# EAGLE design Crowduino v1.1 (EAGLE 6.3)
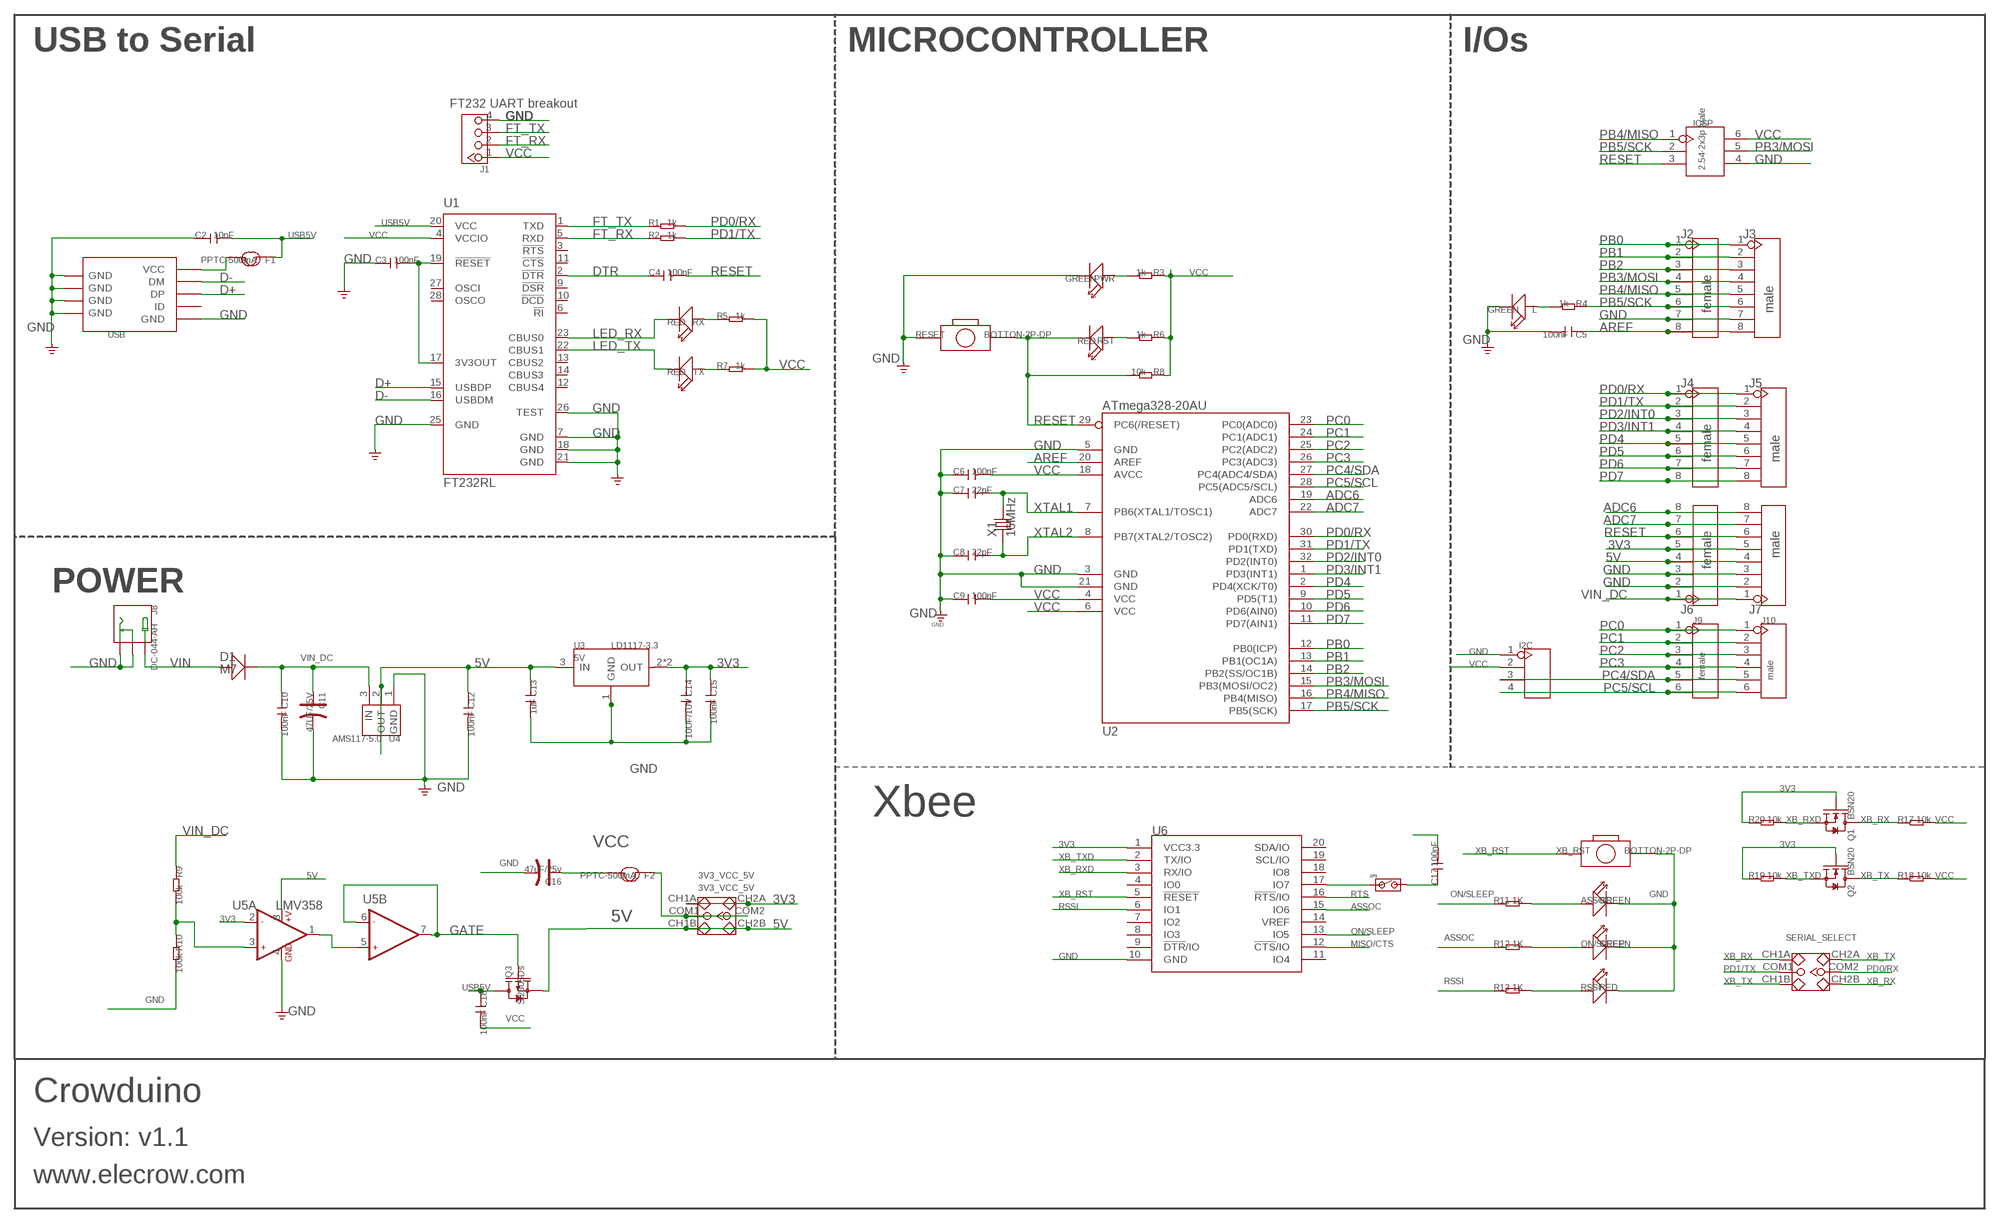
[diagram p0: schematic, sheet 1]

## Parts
3V3_VCC_5V  3V3_VCC_5V  SWITCH-2CH-6P  [6P-2CH-2.54-7.6X3.0]
ASSOC  GREEN  LED'0603'  [LED-0603]
C2  10nF  C-0603  [C0603]
C3  100nF  C-0603  [C0603]
C4  100nF  C-0603  [C0603]
C5  100nF  C-0603  [C0603]
C6  100nF  C-0603  [C0603]
C7  22pF  C-0603  [C0603]
C8  22pF  C-0603  [C0603]
C9  100nF  C-0603  [C0603]
C10  100nF  C-0603  [C0603]
C11  47UF/25V  CAP-ELECTRO-C  [ELECTRO-SMD-C-6MM]
C12  100nF  C-0603  [C0603]
C13  1uF  C-0603  [C0603]
C14  10UF/10V  C-0805  [C0805]
C15  100nF  C-0603  [C0603]
C16  47uF/25v  CAP-ELECTRO-C  [ELECTRO-SMD-C-6MM]
C17  100nF  C-0603  [C0603]
C18  100nF  C-0603  [C0603]
D1  M7  D-SMA  [D2010]
F1  PPTC-500mA  FUSE  [1206@1]
F2  PPTC-500mA  FUSE  [1206@1]
I2C  HEADER-4P-60/35MIL  [4P-65/35MIL]
ICSP  2.54-2x3p male  HEADER-2X3P-2.54  [2X3P-2.54]
J1  CK_1X4_DD  [CK_1X4]
J2  female  HEADER-8P-65/35MIL  [8P-2.54-65/35MIL]
J3  male  HEADER-8P-65/35MIL  [8P-2.54-65/35MIL]
J4  female  HEADER-8P-65/35MIL  [8P-2.54-65/35MIL]
J5  male  HEADER-8P-65/35MIL  [8P-2.54-65/35MIL]
J6  female  HEADER-8P-65/35MIL  [8P-2.54-65/35MIL]
J7  male  HEADER-8P-65/35MIL  [8P-2.54-65/35MIL]
J8  DC-044-AH  DC-044  [DC-404]
J9  female  HEADER-6P-65/35MIL  [6P-2.54-65/35MIL]
J10  male  HEADER-6P-65/35MIL  [6P-2.54-65/35MIL]
JP1  CPT_SMD_JP_SW  [CPT_SMD_JP_SW]
L  GREEN  LED'0603'  [LED-0603]
ON/SLEEP  GREEN  LED'0603'  [LED-0603]
PWR  GREEN  LED'0603'  [LED-0603]
Q1  BSN20  MOSFET-N'SOT23'  [SOT23]
Q2  BSN20  MOSFET-N'SOT23'  [SOT23]
Q3  Si2305Ds  MOSFET-P'SI2323CDS/SI2305DS<BR>'  [SOT23@1]
R1  1k  R-0603  [R0603]
R2  1k  R-0603  [R0603]
R3  1k  R-0603  [R0603]
R4  1k  R-0603  [R0603]
R5  1k  R-0603  [R0603]
R6  1k  R-0603  [R0603]
R7  1k  R-0603  [R0603]
R8  10k  R-0603  [R0603]
R9  100k  R-0603  [R0603]
R10  100k  R-0603  [R0603]
R11  1K  R-0603  [R0603]
R12  1K  R-0603  [R0603]
R13  1K  R-0603  [R0603]
R17  10k  R-0603  [R0603]
R18  10k  R-0603  [R0603]
R19  10k  R-0603  [R0603]
R20  10k  R-0603  [R0603]
RESET  BOTTON-2P-DP  BOTTON-2P-90D  [2P-7.62X3.56-90D]
RSSI  RED  LED'0603'  [LED-0603]
RST  RED  LED'0603'  [LED-0603]
RX  RED  LED'0603'  [LED-0603]
SERIAL_SELECT  3V3_VCC_5V  SWITCH-2CH-6P  [6P-2CH-2.54-7.6X3.0]
TX  RED  LED'0603'  [LED-0603]
U1  FT232RL  [SSOP28]
U2  ATmega328-20AU  ATMEGA168  [TQFP32]
U3  LD1117-3.3  LD1117'SOT89'  [SOT89]
U4  AMS117-5.0  AMS1117SOT223  [SOT-223@1]
U5  LMV358  [SO08]
U6  BEE-OPENBEE  [20-DIP-2.0-W/-SILK]
USB  USB-MINIUSB-5P-STRONG  [MINI-SMD-5P]
X1  16MHz  CRYSTAL-HC49S  [HC49/S]
XB_RST  BOTTON-2P-DP  BOTTON-2P-90D  [2P-7.62X3.56-90D]

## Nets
3V3: 3V3_VCC_5V.CH1A 3V3_VCC_5V.CH2A C14.1 C15.1 J6.5 J7.5 Q1.1(G) Q2.1(G) R19.1 R20.1 U3.2(OUT) U3.4(OUT) U5.2(A:-IN1) U6.1(VCC3.3)
5V [usbvcc]: 3V3_VCC_5V.CH1B 3V3_VCC_5V.CH2B C12.1 C13.1 J6.4 J7.4 Q3.2(S) U3.3(IN) U4.2(OUT) U4.TER(TAB) U5.8(A:+V)
ADC6: J6.8 J7.8 U2.19(ADC6)
ADC7: J6.7 J7.7 U2.22(ADC7)
AREF: C5.1 J2.8 J3.8 U2.20(AREF)
ASSOC: R12.1 U6.15(IO6)
D+: U1.15(USBDP) USB.3(DP)
D-: U1.16(USBDM) USB.2(DM)
DTR: C4.1 U1.2(!DTR)
FT_RX: J1.2 R2.1 U1.5(RXD)
FT_TX: J1.3 R1.1 U1.1(TXD)
GATE: Q3.1(G) U5.6(B:-IN2) U5.7(B:OUT2)
GND: ASSOC.- C2.1 C3.1 C5.2 C6.1 C7.1 C8.1 C9.1 C10.2 C11.- C12.2 C13.2 C14.2 C15.2 C16.- I2C.1 ICSP.4 J1.4 J2.7 J3.7 J6.2 J6.3 J7.2 J7.3 J8.- J8.CDN L.- ON/SLEEP.- PWR.- R10.2 RESET.P$1 RSSI.- U1.7(GND) U1.18(GND) U1.21(GND) U1.25(GND) U1.26(TEST) U2.3(GND) U2.5(GND) U2.21(GND) U3.1(GND) U4.1(GND) U5.4(A:GND) U6.10(GND) USB.5(GND) USB.GND@1(GND) USB.GND@2(GND) USB.GND@3(GND) USB.GND@4(GND) XB_RST.P$2
LED_RX: RX.- U1.23(CBUS0)
LED_TX: TX.- U1.22(CBUS1)
MISO/CTS: U6.12(!CTS!/IO)
N$1: U5.1(A:OUT1) U5.5(B:+IN2)
N$2: F1.2 USB.1(VCC)
N$3: L.+ R4.2
N$4: 3V3_VCC_5V.COM1 3V3_VCC_5V.COM2 F2.1
N$5: JP1.1 U6.17(IO7)
N$6: C3.2 U1.17(3V3OUT) U1.19(!RESET)
N$7: PWR.+ R3.2
N$8: C17.1 JP1.2
N$9: R13.2 RSSI.+
N$11: ON/SLEEP.+ R12.2
N$12: ASSOC.+ R11.2
N$14: R9.2 R10.1 U5.3(A:+IN1)
N$17: R6.2 RST.+
N$31: R5.1 RX.+
N$32: R7.1 TX.+
ON/SLEEP: R11.1 U6.13(IO5)
PB0: J2.1 J3.1 U2.12(PB0(ICP))
PB1: J2.2 J3.2 U2.13(PB1(OC1A))
PB2: J2.3 J3.3 U2.14(PB2(SS/OC1B))
PB3/MOSI: ICSP.5 J2.4 J3.4 U2.15(PB3(MOSI/OC2))
PB4/MISO: ICSP.1 J2.5 J3.5 U2.16(PB4(MISO))
PB5/SCK: ICSP.2 J2.6 J3.6 R4.1 U2.17(PB5(SCK))
PC0: J9.1 J10.1 U2.23(PC0(ADC0))
PC1: J9.2 J10.2 U2.24(PC1(ADC1))
PC2: J9.3 J10.3 U2.25(PC2(ADC2))
PC3: J9.4 J10.4 U2.26(PC3(ADC3))
PC4/SDA: I2C.3 J9.5 J10.5 U2.27(PC4(ADC4/SDA))
PC5/SCL: I2C.4 J9.6 J10.6 U2.28(PC5(ADC5/SCL))
PD0/RX: J4.1 J5.1 R1.2 SERIAL_SELECT.COM2 U2.30(PD0(RXD))
PD1/TX: J4.2 J5.2 R2.2 SERIAL_SELECT.COM1 U2.31(PD1(TXD))
PD2/INT0: J4.3 J5.3 U2.32(PD2(INT0))
PD3/INT1: J4.4 J5.4 U2.1(PD3(INT1))
PD4: J4.5 J5.5 U2.2(PD4(XCK/T0))
PD5: J4.6 J5.6 U2.9(PD5(T1))
PD6: J4.7 J5.7 U2.10(PD6(AIN0))
PD7: J4.8 J5.8 U2.11(PD7(AIN1))
RESET: C4.2 C17.2 ICSP.3 J6.6 J7.6 R8.2 RESET.P$2 RST.- U2.29(PC6(/RESET))
RSSI: R13.1 U6.6(IO1)
RTS: U6.16(!RTS!/IO)
USB5V: C2.2 C18.1 F1.1 Q3.3(D) U1.20(VCC)
VCC: C6.2 C9.2 C16.+ C18.2 F2.2 I2C.2 ICSP.6 J1.1 R3.1 R5.2 R6.1 R7.2 R8.1 R17.2 R18.2 U1.4(VCCIO) U2.4(VCC) U2.6(VCC) U2.18(AVCC)
VIN: D1.+ J8.+
VIN_DC: C10.1 C11.+ D1.- J6.1 J7.1 R9.1 U4.3(IN)
XB_RST: U6.5(!RESET) XB_RST.P$1
XB_RX: Q1.3(D) R17.1 SERIAL_SELECT.CH1A SERIAL_SELECT.CH2B
XB_RXD: Q1.2(S) R20.2 U6.3(RX/IO)
XB_TX: Q2.3(D) R18.1 SERIAL_SELECT.CH1B SERIAL_SELECT.CH2A
XB_TXD: Q2.2(S) R19.2 U6.2(TX/IO)
XTAL1: C7.2 U2.7(PB6(XTAL1/TOSC1)) X1.2
XTAL2: C8.2 U2.8(PB7(XTAL2/TOSC2)) X1.1
Unconnected: U1.3(!RTS) U1.6(!RI) U1.9(!DSR) U1.10(!DCD) U1.11(!CTS) U1.12(CBUS4) U1.13(CBUS2) U1.14(CBUS3) U1.27(OSCI) U1.28(OSCO) U6.4(IO0) U6.7(IO2) U6.8(IO3) U6.9(!DTR!/IO) U6.11(IO4) U6.14(VREF) U6.18(IO8) U6.19(SCL/IO) U6.20(SDA/IO) USB.4(ID)

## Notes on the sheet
- USB to Serial | MICROCONTROLLER | I/Os
- FT232 UART breakout
- POWER
- Xbee
- Crowduino
- Version: v1.1
- www.elecrow.com

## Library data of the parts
3V3_VCC_5V SERIAL_SELECT = Discrete:SWITCH-2CH-6P
ASSOC L ON/SLEEP PWR RSSI RST RX TX = Discrete:LED*
C2-C10 C12-C15 C17 C18 = Discrete:C*: Ceramic Capacitors
C11 C16 = Discrete:CAP*: Electrolytic Capacitors,Tantalum Capacitors and Super Capacitors
D1 = Discrete:D*
F1 F2 = Discrete:FUSE
I2C = Connector:HEADER-4P
ICSP = Connector:HEADER-2X3P
J1 = CONNECTER:CK_1X4
J2-J7 = Connector:HEADER-8P
J8 = For_Test_Albert:DC-044
J9 J10 = Connector:HEADER-6P
JP1 = Elecrow_test:CPT_SMD_JP_SW
Q1 Q2 = Discrete:MOSFET-N: IRLL014: http://www.vishay.com/docs/91319/sihll014.pdf
Q3 = Discrete:MOSFET-P
R1-R13 R17-R20 = Discrete:R*
RESET XB_RST = Discrete:BOTTON-2P
U1 = IC_SMD:FT232R: Source: http://www.ftdichip.com/Documents/DataSheets/DS_FT232R_v104.pdf
U2 = IC:ATMEGA168
U3 = IC:LD1117: Low Drop Fixed And Adjustable Positive Voltage Regulators http://www.datasheetcatalog.org/datasheet/SGSThomsonMicroelectronics/mXuqtqv.pdf
U4 = IC:AMS1117
U5 = IC:LMV358
U6 = moudle:BEE-OPENBEE
USB = Connector:USB-MINIUSB-5P
X1 = Discrete:CRYSTAL*: CRYSTAL

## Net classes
0 default: clearance 0.152 mm
1 power: width 0.203 mm, drill 0.305 mm, clearance 0.203 mm
2 gnd: width 0.203 mm, drill 0.305 mm, clearance 0.203 mm
3 usbvcc: width 0.203 mm, drill 0.305 mm, clearance 0.203 mm

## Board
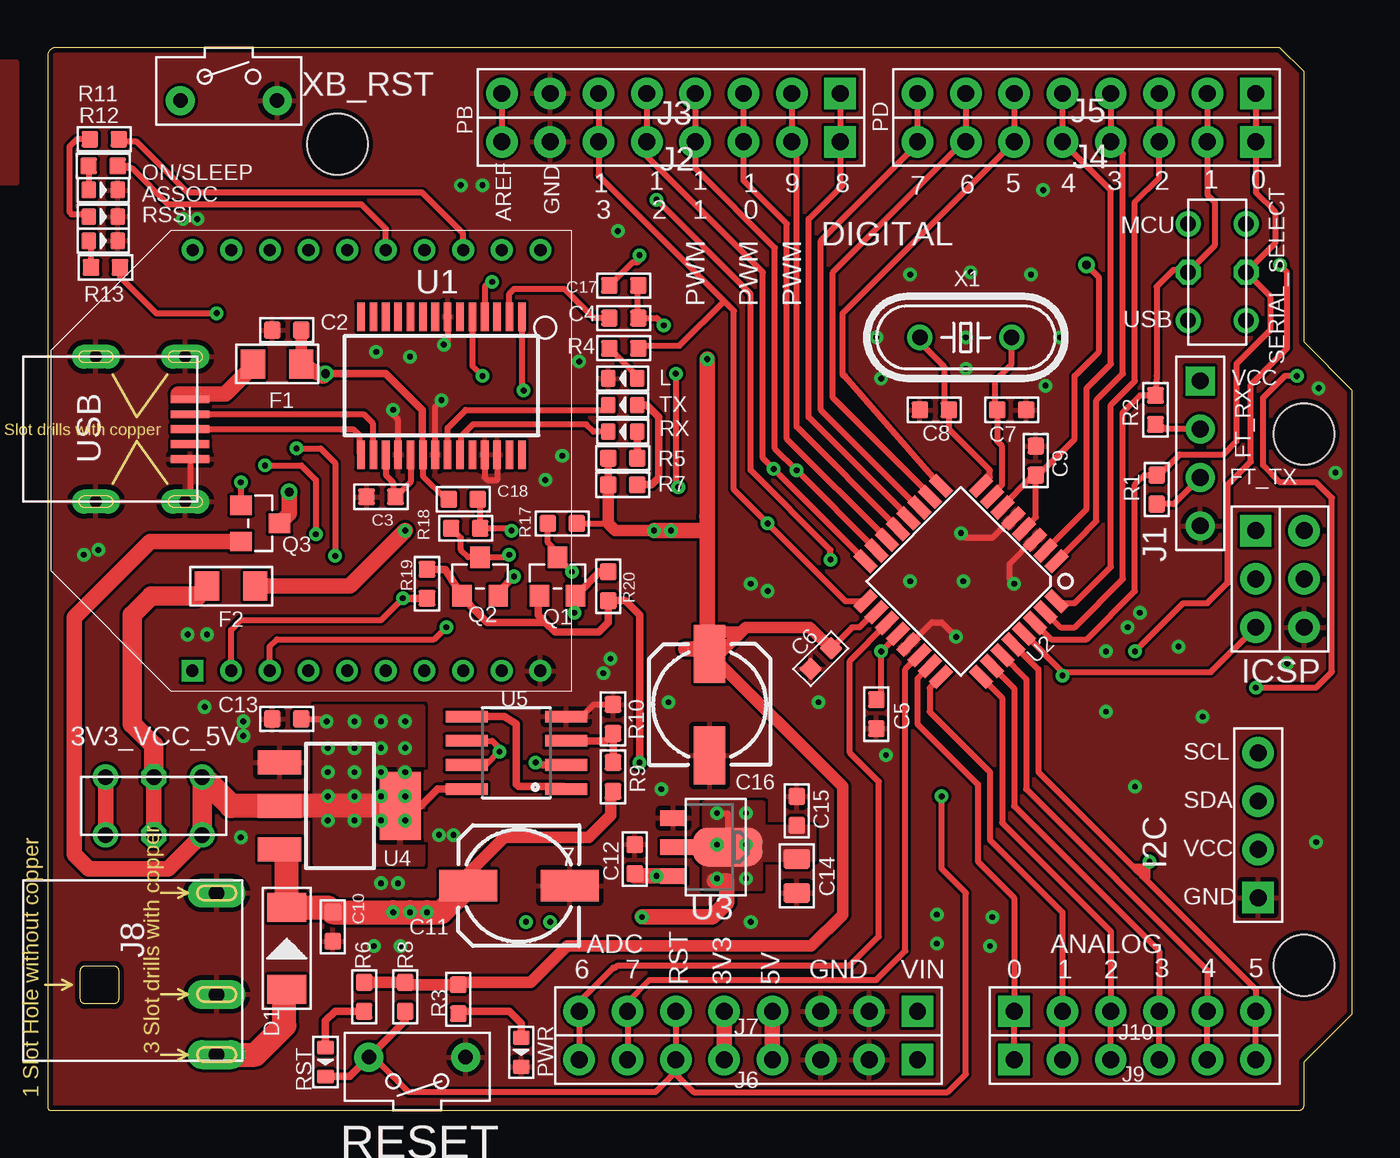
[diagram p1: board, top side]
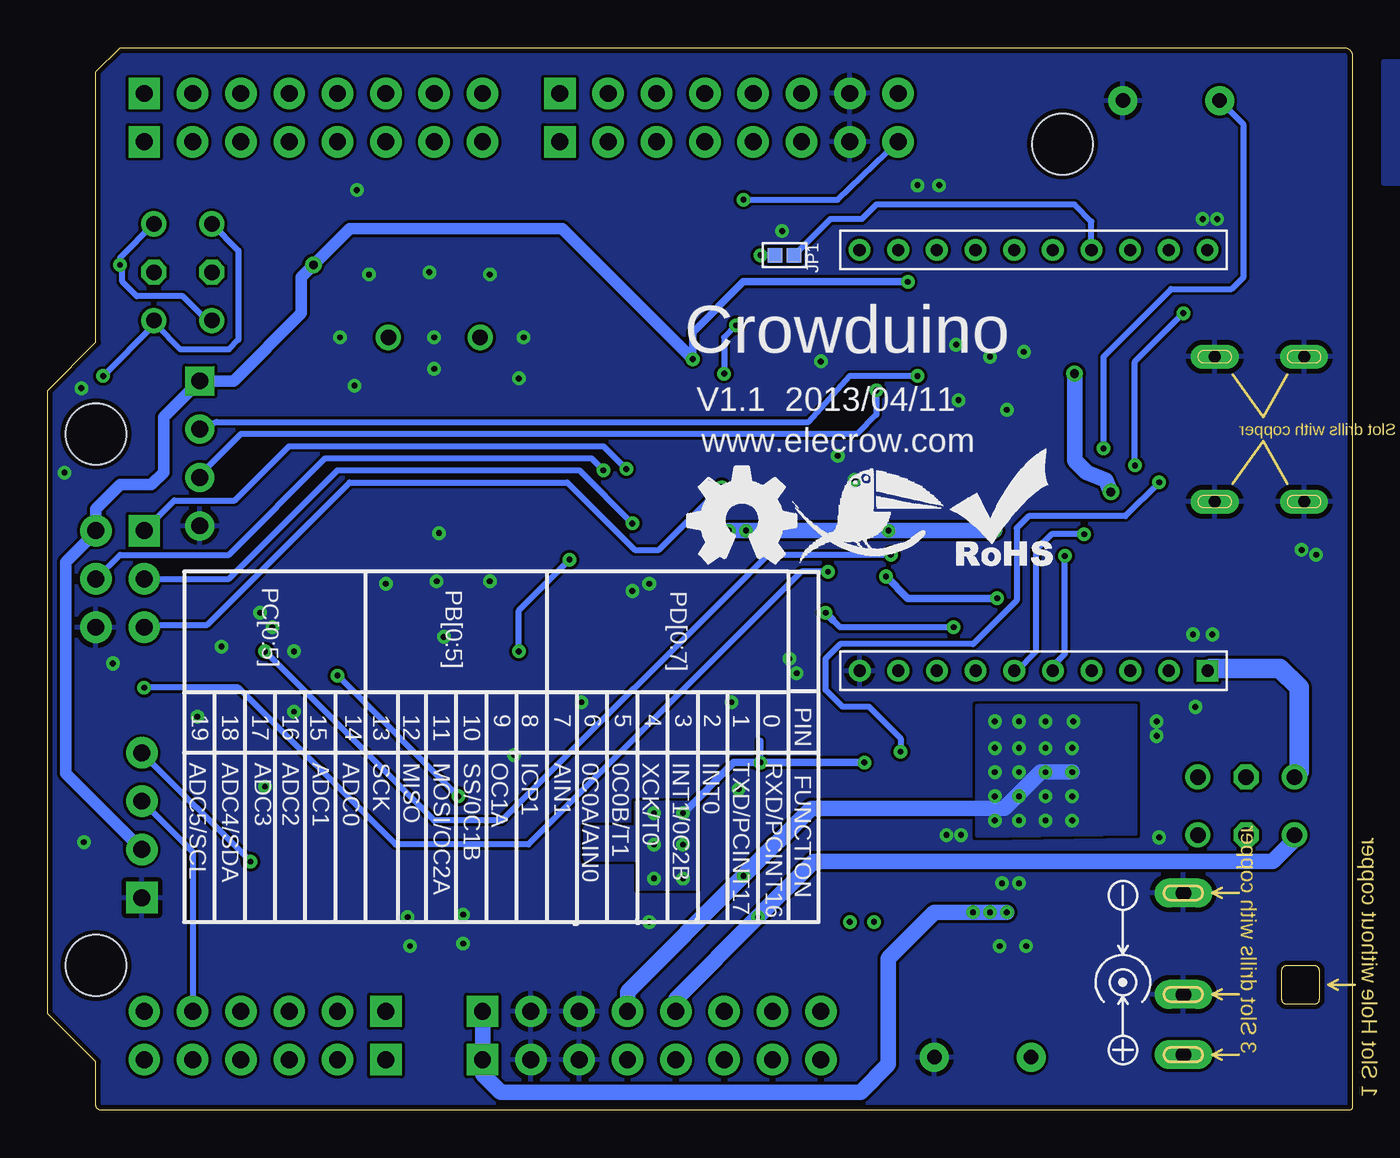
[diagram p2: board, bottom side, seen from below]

Size 68.58 x 55.88 mm. Coordinates in mm from the lower left corner, seen from the top.
Outline: 64.77,55.88 0.46,55.88 arc90 0,55.42 0,0.18 arc90 0.18,0 65.76,0 arc90 66.04,0.28 66.04,2.54 68.58,5.08 68.58,37.85 66.04,40.39 66.04,54.61 64.77,55.88
Copper layers (1*16): Top 0.035mm / dielectric 1.5mm / Bottom 0.035mm
Design rules "default *": minimum track width 10mil, minimum drill 12mil, track to track 6mil, track to pad 6mil, pad to pad 6mil, via to via 10mil, smd to smd 0mil, copper to edge 10mil, drill to drill 10mil, minimum pad ring 10mil, minimum via ring 8mil, stop-mask expansion 2mil, vias tented up to drill 25mil, thermal gap 10mil
Holes 3.2 mm at 66.04,7.62 66.04,35.56 15.24,50.8

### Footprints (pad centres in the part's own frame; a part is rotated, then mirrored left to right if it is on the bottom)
6P-2CH-2.54-7.6X3.0 = drill 0.813 pad 1.27: CH1A -1.524,2.54; CH1B -1.524,-2.54; CH2A 1.524,2.54; CH2B 1.524,-2.54 | drill 0.813 pad 1.27 octagon: COM1 -1.524,0; COM2 1.524,0
LED-0603 = smd 0.762 x 0.889: + -0.762,0; - 0.762,0
C0603 = smd 0.889 x 0.889: 1 -0.762,0; 2 0.762,0
ELECTRO-SMD-C-6MM = smd 3.048 x 1.651: + 2.667,0; - -2.667,0
C0805 = smd 1.016 x 1.397: 1 -0.889,0; 2 0.889,0
D2010 = smd 1.524 x 2.032: + -2.159,0; - 2.159,0
1206@1 = smd 1.27 x 1.524: 1 -1.27,0; 2 1.27,0
4P-65/35MIL = drill 0.889 pad 1.651 square: 1 0,3.81 | drill 0.889 pad 1.651: 2 0,1.27; 3 0,-1.27; 4 0,-3.81
2X3P-2.54 = drill 0.889 pad 1.651 square: 1 -1.27,2.54 | drill 0.889 pad 1.651: 2 -1.27,0; 3 -1.27,-2.54; 4 1.27,-2.54; 5 1.27,0; 6 1.27,2.54
CK_1X4 = drill 0.889 pad 1.524 square: 1 0,3.81 | drill 0.889 pad 1.524: 2 0,1.27; 3 0,-1.27; 4 0,-3.81
8P-2.54-65/35MIL = drill 0.889 pad 1.651 square: 1 0,8.89 | drill 0.889 pad 1.651: 2 0,6.35; 3 0,3.81; 4 0,1.27; 5 0,-1.27; 6 0,-3.81; 7 0,-6.35; 8 0,-8.89
DC-404 = drill 0.813 pad 1.524 long: + 3.175,10.16; - -5.334,10.16; CDN 0,10.16
6P-2.54-65/35MIL = drill 0.889 pad 1.651 square: 1 0,6.35 | drill 0.889 pad 1.651: 2 0,3.81; 3 0,1.27; 4 0,-1.27; 5 0,-3.81; 6 0,-6.35
CPT_SMD_JP_SW = smd 0.762 x 0.762: 1 0,0.508; 2 0,-0.508
SOT23 = smd 1.016 x 1.143: 1 -0.95,-1.016; 2 0.95,-1.016; 3 0,1.016
SOT23@1 = smd 1.016 x 1.143: 1 -0.95,-1.016; 2 0.95,-1.016; 3 0,1.016
R0603 = smd 0.889 x 0.889: 1 -0.762,0; 2 0.762,0
2P-7.62X3.56-90D = drill 0.762 pad 1.524: P$1 0,2.54; P$2 0,-2.54
SSOP28 = smd 0.4 x 1.5: 1 -4.225,-3.625; 2 -3.575,-3.625; 3 -2.925,-3.625; 4 -2.275,-3.625; 5 -1.625,-3.625; 6 -0.975,-3.625; 7 -0.325,-3.625; 8 0.325,-3.625; 9 0.975,-3.625; 10 1.625,-3.625; 11 2.275,-3.625; 12 2.925,-3.625; 13 3.575,-3.625; 14 4.225,-3.625; 15 4.225,3.625; 16 3.575,3.625; 17 2.925,3.625; 18 2.275,3.625; 19 1.625,3.625; 20 0.975,3.625; 21 0.325,3.625; 22 -0.325,3.625; 23 -0.975,3.625; 24 -1.625,3.625; 25 -2.275,3.625; 26 -2.925,3.625; 27 -3.575,3.625; 28 -4.225,3.625
TQFP32 = smd 1.27 x 0.559: 1 -4.293,2.8; 2 -4.293,2; 3 -4.293,1.2; 4 -4.293,0.4; 5 -4.293,-0.4; 6 -4.293,-1.2; 7 -4.293,-2; 8 -4.293,-2.8; 17 4.293,-2.8; 18 4.293,-2; 19 4.293,-1.2; 20 4.293,-0.4; 21 4.293,0.4; 22 4.293,1.2; 23 4.293,2; 24 4.293,2.8 | smd 0.559 x 1.27: 9 -2.8,-4.293; 10 -2,-4.293; 11 -1.2,-4.293; 12 -0.4,-4.293; 13 0.4,-4.293; 14 1.2,-4.293; 15 2,-4.293; 16 2.8,-4.293; 25 2.8,4.293; 26 2,4.293; 27 1.2,4.293; 28 0.4,4.293; 29 -0.4,4.293; 30 -1.2,4.293; 31 -2,4.293; 32 -2.8,4.293
SOT89 = smd 0.8 x 1.4: 1 -1.524,-1.905; 3 1.524,-1.905 | smd 0.8 x 1.9: 2 0,-1.651 | smd 2.032 x 3.65: 4 0,0.94
SOT-223@1 = smd 1.27 x 2.286: 1 -2.286,-3.175; 2 0,-3.175; 3 2.286,-3.175 | smd 3.556 x 2.159: TER 0,3.175
SO08 = smd 0.61 x 2.21: 1 -1.905,-2.616; 2 -0.635,-2.616; 3 0.635,-2.616; 4 1.905,-2.616; 5 1.905,2.616; 6 0.635,2.616; 7 -0.635,2.616; 8 -1.905,2.616
20-DIP-2.0-W/-SILK = drill 0.635 pad 1.016 square: 1 0,0.008 | drill 0.635 pad 1.016: 2 0,-2.024; 3 0,-4.056; 4 0,-6.088; 5 0,-8.12; 6 0,-10.152; 7 0,-12.184; 8 0,-14.216; 9 0,-16.248; 10 0,-18.28; 11 22.123,-18.288; 12 22.123,-16.256; 13 22.123,-14.224; 14 22.123,-12.192; 15 22.123,-10.16; 16 22.123,-8.128; 17 22.123,-6.096; 18 22.123,-4.064; 19 22.123,-2.032; 20 22.123,0
MINI-SMD-5P = smd 2.032 x 0.406: 1 0.381,-1.575; 2 0.381,-0.787; 3 0.381,0; 4 0.381,0.787; 5 0.381,1.575 | drill 0.635 pad 1.27 long: GND@1 0.635,3.81; GND@2 5.334,3.81; GND@3 5.334,-3.81; GND@4 0.635,-3.81
HC49/S = drill 0.813: 1 -2.413,0; 2 2.413,0

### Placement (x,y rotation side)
3V3_VCC_5V  5.59,16 90 top
ASSOC  2.92,46.99 0 top
C2  12.57,41.02 0 top
C3  17.53,32.26 0 top
C4  30.29,41.66 0 top
C5  43.56,20.83 270 top
C6  40.64,23.75 45 top
C7  50.67,36.83 180 top
C8  46.61,36.83 0 top
C9  51.94,34.16 270 top
C10  14.99,9.65 270 top
C11  24.77,11.81 180 top
C12  30.86,13.21 90 top
C13  12.57,20.57 180 top
C14  39.37,12.32 270 top
C15  39.37,15.75 90 top
C16  34.8,21.34 90 top
C17  30.29,43.37 0 top
C18  21.84,32.13 0 top
D1  12.57,8.51 90 top
F1  12.06,39.24 180 top
F2  9.65,27.56 0 top
I2C  63.63,14.99 180 top
ICSP  64.77,27.94 0 top
J1  60.58,34.54 0 top
J2  32.77,50.93 270 top
J3  32.77,53.47 270 top
J4  54.61,50.93 270 top
J5  54.61,53.47 270 top
J6  36.83,2.67 270 top
J7  36.83,5.21 270 top
J8  -1.27,6.1 270 top
J9  57.15,2.67 90 top
J10  57.15,5.21 90 top
JP1  29.84,44.96 270 bottom
L  30.23,38.48 180 top
ON/SLEEP  2.92,48.39 0 top
PWR  24.89,3.05 270 top
Q1  26.8,28.07 0 top
Q2  22.73,28.07 0 top
Q3  11.18,30.86 270 top
R1  58.29,32.64 90 top
R2  58.23,36.83 90 top
R3  21.59,5.84 270 top
R4  30.29,40.07 180 top
R5  30.23,34.29 180 top
R6  16.64,5.97 270 top
R7  30.23,32.89 180 top
R8  18.8,5.97 270 top
R9  29.72,17.53 90 top
R10  29.72,20.57 90 top
R11  2.98,51.05 180 top
R12  2.92,49.66 180 top
R13  3.05,44.32 180 top
R17  27.05,30.86 0 top
R18  21.97,30.61 0 top
R19  19.94,27.69 270 top
R20  29.46,27.56 90 top
RESET  19.43,2.79 270 top
RSSI  2.92,45.72 0 top
RST  14.61,2.54 270 top
RX  30.23,35.69 180 top
SERIAL_SELECT  61.47,44.07 0 top
TX  30.23,37.08 180 top
U1  20.7,38.1 180 top
U2  48.01,27.81 225 top
U3  34.8,13.84 270 top
U4  15.37,16 270 top
U5  24.64,18.8 90 top
U6  7.62,23.11 90 top
U$1  [OSHW_FILLX200_NOTEXT]  34.92,28.77 0 bottom
U$2  [ELECROW4]  30.23,27.37 0 bottom
U$3  [ROHS_SILK]  19.05,31.05 0 bottom
USB  7.87,35.81 180 top
X1  48.26,40.64 0 top
XB_RST  9.53,53.09 90 top

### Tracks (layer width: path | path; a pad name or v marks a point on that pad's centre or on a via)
3V3  (via drill 0.3)
  Top 0.305: C14.1 39.37,13.27 39.43,13.21 | 39.37,15.24 C15.1 | v35.18,15.62 35.74,15.62 U3.4
  Top 0.406: v31.11,18.29 31.11,26.04 30.35,26.8 R20.1 | 26.16,25.65 25.78,26.04 25.78,26.98 Q1.1 | R19.1 20.89,28.45 Q2.1 22.29,26.48 23.11,25.65 26.16,25.65 | 26.16,25.65 26.67,25.15 28.96,25.15 29.46,25.65 R20.1 | 29.72,26.54 R20.1 | U5.2 26.04,18.16 v25.65,18.29
  Top 0.813: 3V3_VCC_5V.CH2A 3V3_VCC_5V.CH1A | U3.2 35.18,13.84 | v31.24,10.16 34.92,10.16 35.69,10.92 35.69,12.06 35.05,12.06 | J6.5 J7.5
  Bottom 0.305: 31.11,19.43 v31.11,18.29
  Bottom 0.406: v25.65,18.29 v31.11,18.29 32.51,18.29 v35.18,15.62
  Bottom 0.813: 3V3_VCC_5V.CH1A 3.05,14.22 4.19,13.08 28.32,13.08 v31.24,10.16 35.56,5.84 J7.5
  Bottom 1.016: 3V3_VCC_5V.CH2A 2.79,17.78 2.79,22.23 3.81,23.24 7.49,23.24 U6.1
  other vias: 35.18,13.97 35.18,12.19 36.7,12.19 36.7,15.62 36.7,13.97
  pour Bottom (isolate 0.254, no thermals): 34.54,16.13 34.54,11.68 37.47,11.68 37.47,13.21 40.26,13.21 40.26,14.86 37.59,14.86 37.59,16.13
  pour Top (isolate 0.254, no thermals): 34.54,16.13 34.54,11.68 37.47,11.68 37.47,13.21 40.26,13.21 40.26,14.86 37.59,14.86 37.59,16.13
5V  (via drill 0.3)
  Top 0.305: C13.1 14.54,20.57 v14.67,20.45
  Top 0.406: U5.8 21.89,16.76 21.77,16.89 20.51,16.89 19.62,16 U4.TER
  Top 0.813: U3.3 v32,12.32 30.99,12.32 | 30.86,12.32 30.99,12.32 | C12.1 30.99,12.32 | 3V3_VCC_5V.CH1B 6.35,12.7 2.16,12.7 1.4,13.46 1.4,25.91 5.4,29.91 Q3.2 | J6.4 J7.4
  Top 1.016: 3V3_VCC_5V.CH2B 3V3_VCC_5V.CH1B
  Top 1.27: U4.TER U4.2 9.65,16 3V3_VCC_5V.CH2B
  Bottom 0.813: v14.73,17.78 v16.13,17.78 16.38,17.78 18.29,15.88 28.45,15.88 v32,12.32 38.1,6.22 J7.4
  other vias: 14.73,19.05 16.13,19.05 17.53,19.05 18.8,19.05 18.8,20.45 17.53,20.45 16.13,20.45 14.73,15.24 16.13,15.24 14.73,16.51 16.13,16.51 17.53,17.78 18.8,17.78 17.53,16.51 18.8,16.51 17.53,15.24 18.8,15.24
  pour Bottom: 11.43,14.61 11.43,21.21 19.68,21.21 19.68,14.48
  pour Top: 14.1,21.21 19.68,21.21 19.68,12.95 14.1,12.95
ADC6
  Top 0.305: U2.19 42.16,23.62 42.16,18.8 43.69,17.27 43.69,9.14 42.16,7.62 29.97,7.62 29.84,7.49 29.72,7.49 27.94,5.71 J7.8 J6.8
ADC7
  Top 0.305: U2.22 45.09,23.2 45.09,8.38 43.56,6.86 31.62,6.86 30.48,5.71 J7.7 J6.7
AREF  (via drill 0.3)
  Top 0.305: C5.1 43.81,21.84 v43.81,24.13 44.69,25 U2.20 | v41.15,28.96 41.15,29.46 36.96,33.66 36.96,42.93 v32,47.88 | J3.8 J2.8
  Bottom 0.305: v43.81,24.13 43.81,26.29 v41.15,28.96 | v32,47.88 27.05,47.88 J2.8
ASSOC
  Top 0.305: 4.19,49.66 R12.1 3.94,49.53 4.45,49.53 6.35,47.62 16.51,47.62 17.78,46.35 U6.15
D+
  Top 0.305: USB.3 16.07,35.81 16.38,35.5 16.38,34.57 U1.15
D-
  Top 0.305: USB.2 16.61,36.6 17.08,36.13 17.08,34.52 U1.16
DTR
  Top 0.305: U1.2 24.28,42.95 24.51,43.18 27.18,43.18 28.7,41.66 C4.1
FT_RX  (via drill 0.3)
  Top 0.305: J1.2 58.8,35.81 R2.1 | U1.5 22.33,39.14 v22.86,38.61
  Bottom 0.305: J1.2 60.58,35.94 59.69,36.2 28.57,36.2 26.42,38.61 v22.86,38.61
FT_TX  (via drill 0.3)
  Top 0.305: J1.3 59.18,31.88 R1.1 | U1.1 24.93,37.94 v25.02,37.85
  Bottom 0.305: J1.3 60.58,33.4 58.42,35.56 26.04,35.56 25.02,36.58 v25.02,37.85
GATE  (via drill 0.3)
  Top 0.305: v10.16,33.02 Q3.1 | U5.6 23.37,19.43 23.75,19.05 v23.75,18.86 23.05,18.16 U5.7
  Bottom 0.305: v23.75,18.86 23.75,19.56 25.4,21.21 26.8,21.21 27.69,22.1 27.69,23.75 26.92,24.51 19.94,24.51 17.65,26.8 17.65,30.61 17.02,31.24 11.94,31.24 v10.16,33.02
GND  (via drill 0.3)
  Top 0.305: U5.4 28.07,20.7 28.7,21.34 R10.2 | U2.21 45.32,24.5 46.48,25.65 46.99,25.65 v47.75,24.89 | U2.3 51.84,30 50.55,28.7 50.55,27.94 v50.8,27.69 | U2.5 50.69,31.13 49.66,30.1 48.26,30.1 v48.01,30.35 | U1.7 21.03,40.46 v20.83,40.26 | U1.21 20.38,37.01 v20.7,37.34 | U1.18 18.43,36.31 18.16,36.58 v18.16,36.83 | U1.26 23.63,33.15 23.62,33.15 23.11,33.15 22.98,33.28 U1.25 | USB.5 7.49,32.26 USB.GND@1
  other vias: 46.74,10.29 46.74,8.76 49.66,10.16 49.53,8.64 52.32,48.39 48.51,44.07 48.26,40.64 48.26,38.99 43.56,40.64 53.21,40.64 45.34,27.81 60.71,20.7 21.34,14.48 10.16,14.35 10.29,20.45 2.67,29.46 1.91,29.21 19.05,39.62 10.29,19.68 17.27,39.88 8.26,21.21 36.96,27.69 48.13,27.81 18.41,11.94 17.53,11.94 20.57,14.48 57.15,17.02 36.96,9.91 32.26,16.89 55.63,20.95 17.14,8.64 18.54,8.64 7.11,46.86 7.87,46.86 43.81,38.48 52.45,38.1 40.51,21.46 44.07,18.67 29.97,46.23 37.85,27.3 21.72,48.64 22.86,48.64 65.15,23.5 57.4,26.16 56.77,25.4 51.69,43.94 45.34,43.94 7.37,25.02 8.38,25.02 29.21,22.99 59.44,24.38 32.64,21.46 29.59,23.75 55.63,24.13 67.69,33.53 66.8,37.97 66.67,14.1 27.94,39.37 27.05,34.42 26.16,33.15
  pour Top: -8.64,55.12 -1.65,55.12 -1.65,48.77 -8.64,48.77 -8.64,48.9
  pour Bottom (rank 6): -8.64,55.12 -1.65,55.12 -1.65,48.77 -8.76,48.77 -8.76,48.9 -8.64,48.9
  pour Top (rank 6): 0,0 68.58,0 68.58,55.88 0,55.88
  pour Bottom (rank 6): 0,0 68.58,0 68.58,38.1 68.58,55.88 0,55.88
LED_RX
  Top 0.305: RX.- 28.7,35.69 28.32,36.07 22.35,36.07 21.72,35.43 21.72,34.52 U1.23
LED_TX
  Top 0.305: U1.22 21.03,35.88 21.97,36.83 29.21,36.83 TX.-
N$1
  Top 0.406: U5.5 24,20.7 24.64,20.32 24.64,17.14 24.77,17.02 27.13,17.02 U5.1
N$2
  Top 0.305: 6.86,37.66 7.04,37.85 USB.1
  Top 0.813: F1.2 10.67,39.24 10.67,38.99 9.34,37.66 6.86,37.66
N$3
  Top 0.305: R4.2 30.99,38.61 L.+
N$4
  Top 0.813: 3V3_VCC_5V.COM2 3V3_VCC_5V.COM1
  Top 1.016: 3V3_VCC_5V.COM2 5.59,19.18 4.45,20.32 4.45,26.04 5.46,27.05 7.87,27.05 F2.1
N$5
  Bottom 0.305: U6.17 13.72,46.74 14.61,47.62 25.02,47.62 25.78,46.86 27.43,46.86 JP1.1
N$6
  Top 0.305: U1.17 17.78,33.41 18.16,33.02 18.16,32.38 C3.2 19.08,33.05 U1.19
N$7
  Top 0.406: PWR.+ 24.89,4.57 24.26,5.21 21.72,5.21 R3.2
N$8  (via drill 0.3)
  Top 0.305: v31.11,44.96 31.11,44.7 30.99,44.58 30.73,44.58 C17.1
  Bottom 0.305: JP1.2 v31.11,44.96
N$9
  Top 0.305: R13.2 2.29,45.59 RSSI.+
N$11
  Top 0.305: R12.2 ON/SLEEP.+
N$12
  Top 0.305: R11.2 1.52,51.05 1.14,50.67 1.14,47.24 1.27,47.12 2.03,47.12 ASSOC.+
N$14
  Top 0.406: 29.59,18.16 R9.2 R10.1 29.34,19.43 U5.3
N$17
  Top 0.406: RST.+ 14.61,4.7 15.11,5.21 R6.2
N$19  (via drill 0.3)
  other vias: 25.15,9.91
N$21  (via drill 0.3)
  other vias: 26.42,9.91
N$31
  Top 0.406: RX.+ R5.1
N$32
  Top 0.406: TX.+ 31.5,37.08 32.13,36.45 32.13,33.27 31.75,32.89 R7.1
ON/SLEEP
  Top 0.305: U6.13 21.84,46.1 19.68,48.26 7.37,48.26 4.7,50.93 3.87,50.93 R11.1
PB0
  Top 0.305: U2.12 45.25,31.2 40.01,36.45 40.01,46.86 41.53,48.39 41.66,48.51 | 41.66,48.51 41.78,48.64 | J3.1 J2.1 41.66,48.51
PB1
  Top 0.305: U2.13 44.69,30.62 39.37,35.94 39.37,50.67 J2.2 J3.2
PB2
  Top 0.305: U2.14 44.12,30.05 38.86,35.31 38.86,46.61 36.58,48.9 J2.3 J3.3
PB3/MOSI  (via drill 0.3)
  Top 0.305: U2.15 43.56,29.47 v39.37,33.66 38.23,34.8 38.23,45.34 34.04,49.53 J2.4 J3.4
  Bottom 0.305: ICSP.5 64.77,29.21 59.05,29.21 53.98,34.29 40.01,34.29 v39.37,33.66
PB4/MISO  (via drill 0.3)
  Top 0.305: U2.16 42.99,28.89 v38.16,33.72 37.59,34.29 37.59,44.07 31.5,50.16 J2.5 J3.5
  Bottom 0.305: ICSP.1 61.91,32.07 58.74,32.07 55.88,34.92 39.37,34.92 v38.16,33.72
PB5/SCK  (via drill 0.3)
  Top 0.305: U2.17 41.95,26.76 v37.85,30.86 36.07,32.64 36.07,42.04 35.56,42.55 | 35.56,42.55 28.96,49.15 J2.6 J3.6 | 35.56,42.55 33.21,40.2 31.05,40.2 R4.1
  Bottom 0.305: ICSP.2 59.05,27.94 53.34,33.66 40.64,33.66 v37.85,30.86
PC0
  Top 0.305: U2.23 45.72,22.7 45.72,20.32 48.9,17.14 48.9,13.08 50.8,11.18 J10.1 J9.1
PC1
  Top 0.305: U2.24 46.35,22.2 46.35,20.95 49.53,17.78 49.53,14.22 53.34,10.41 J10.2 J9.2
PC2
  Top 0.305: U2.25 50.16,21.69 50.16,15.11 55.88,9.4 J10.3 J9.3
PC3
  Top 0.305: U2.26 50.8,22.19 50.8,16 58.42,8.38 J10.4 J9.4
PC4/SDA
  Top 0.305: U2.27 51.44,22.69 51.44,16.89 60.96,7.37 J10.5 J9.5
  Bottom 0.305: I2C.3 60.96,13.59 J10.5
PC5/SCL  (via drill 0.3)
  Top 0.305: U2.28 52.07,23.18 52.07,17.78 57.02,12.83 | 57.02,12.83 57.28,12.57 | 57.28,12.57 57.53,12.32 | 57.53,12.32 63.5,6.35 J10.6 J9.6 | v57.91,13.08 57.4,12.57 57.28,12.57 | 57.53,12.32 57.66,12.45 | 57.66,12.45 57.66,12.57 | 57.66,12.45 57.66,12.32 | 57.02,12.83 57.66,12.83 57.78,12.7 57.78,12.19
  Bottom 0.305: I2C.4 v57.91,13.08
PD0/RX
  Top 0.305: U2.30 52.75,24.77 54.61,24.77 57.15,27.3 57.15,32.89 57.66,33.4 R1.2 58.42,33.4 59.5,34.48 61.78,34.48 62.48,35.18 62.48,39.24 64.26,41.02 64.26,42.8 SERIAL_SELECT.COM2 64.52,45.59 64.52,47.24 63.5,48.26 J4.1 J5.1
PD1/TX
  Top 0.305: U2.31 53.25,25.4 53.98,25.4 56.52,27.94 56.52,36.7 57.4,37.59 R2.2 58.29,38.61 58.29,43.31 59.18,44.2 59.82,44.2 SERIAL_SELECT.COM1 61.34,45.47 61.34,47.75 60.96,48.13 J4.2 J5.2
PD2/INT0
  Top 0.305: U2.32 53.11,26.67 53.98,26.67 55.88,28.57 55.88,37.08 57.15,38.35 57.15,47.75 58.42,49.02 J4.3 J5.3
PD3/INT1
  Top 0.305: U2.1 54.61,30.46 54.61,30.48 55.12,30.99 55.12,37.34 56.52,38.73 56.52,50.29 J4.4 J5.4
PD4
  Top 0.305: U2.2 52.46,29.47 54.61,31.62 54.61,37.97 55.88,39.24 55.88,48.39 J4.5 J5.5
PD5
  Top 0.305: U2.9 46.19,33.69 41.91,38.61 arc-90 41.78,38.73 41.78,41.91 J4.6 J5.6
PD6
  Top 0.305: U2.10 46.38,32.35 41.27,37.47 41.27,44.07 48.13,50.93 J4.7 J5.7
PD7
  Top 0.305: U2.11 45.77,31.7 40.64,36.83 40.64,45.72 45.72,50.8 J4.8 J5.8
RESET  (via drill 0.3)
  Top 0.305: U2.29 53.34,23.05 | 53.34,23.05 61.15,23.05 ICSP.3 | v46.99,16.51 46.99,12.7 48.26,11.43 48.26,1.91 47.31,0.95 33.97,0.95 33.02,1.91 33.02,2.03 | v53.34,22.86 53.34,23.05 | 33.02,2.03 31.94,0.95 18.99,0.95 17.14,2.79 RESET.P$2 | v33.02,38.73 33.02,32.89 v33.15,32.77 | J7.6 J6.6 33.02,2.03 | v32.38,41.27 32,41.66 C4.2 30.99,41.72 30.99,43.31 C17.2
  Top 0.406: RST.- 15.88,1.78 RESET.P$2 18.8,4.7 R8.2
  Bottom 0.305: ICSP.3 63.37,25.53 60.2,25.53 52.7,33.02 41.27,33.02 37.72,29.46 36.45,29.46 v33.15,32.77 | 33.02,38.99 v33.02,38.73 33.02,40.64 v32.38,41.27 | v46.99,16.51 v53.34,22.86 53.34,23.05
RSSI  (via drill 0.3)
  Top 0.305: v8.89,41.91 5.71,41.91 3.81,43.81 R13.1 | v14.1,30.29 14.1,33.15 13.34,33.91 v11.43,33.91
  Bottom 0.305: U6.6 17.65,23.11 16.64,24.13 16.64,29.46 15.81,30.29 v14.1,30.29 | v11.43,33.91 11.43,39.37 v8.89,41.91
USB5V  (via drill 0.46)
  Top 0.305: 19.68,35.6 19.73,35.56 U1.20 19.73,33.36 20.95,32.13 C18.1
  Top 0.406: v14.61,38.73 17.78,38.73 19.68,36.83 19.68,35.6
  Top 0.61: C2.2 F1.1
  Top 0.813: F1.1 14.48,38.61 v14.61,38.73 | v12.7,32.51 12.7,31.37 Q3.3
  Bottom 0.813: v14.61,38.73 14.61,34.16 13.97,33.53 12.95,33.15 v12.7,32.51
VCC  (via drill 0.3, 0.46)
  Top 0.305: 51.14,30.57 U2.4 51.94,31.18 C9.2 52.07,33.4 | U2.6 49.99,31.5 49.91,31.5 51.94,33.53 52.07,33.4 | 52.07,33.4 53.98,35.31 53.98,38.61 55.24,39.88 55.24,43.81 v54.61,44.45 | U2.18 43.46,26.19 42.67,25.4 42.29,25.4 C6.2 | 35.05,25.02 34.8,24.77 C16.+ | U1.4 22.99,43.31 23.24,43.56 | R17.2 29.59,30.86 29.97,30.48 | C18.2 22.73,32 R18.2 24.26,30.61 v24.38,30.48
  Top 0.406: v23.37,43.56 23.24,43.56 | R5.2 R7.2
  Top 0.61: C6.2 40.07,25.4 36.7,25.4 36.45,25.15 | 36.45,25.15 35.31,24 C16.+ | 36.45,25.15 34.67,25.15 | 34.67,24.13 41.78,17.02 41.78,10.29 40.13,8.64 27.3,8.64 25.4,6.73 21.72,6.73 R3.1 18.92,6.6 R8.1 R6.1 | 34.54,31.24 34.67,31.11 | R7.2 29.46,30.86 29.84,30.48 29.97,30.48 v31.88,30.48
  Top 0.813: 34.67,25.15 34.67,30.48 | 34.67,30.48 34.67,31.11 v34.67,39.5 | 34.54,24.26 33.53,24.26 | F2.2 15.88,27.56 v18.8,30.48 | 34.67,30.48 v32.77,30.48 v31.88,30.48
  Top 1.016: 34.54,24.26 34.67,24.13 C16.+
  Bottom 0.406: v23.37,43.56 32,43.56 34.67,40.89 v34.67,39.5
  Bottom 0.61: v34.67,39.5 41.53,46.35 52.7,46.35 v54.61,44.45 55.24,43.81 55.24,41.91 58.8,38.35 J1.1 62.48,36.45 62.48,33.53 63.12,32.89 64.77,32.89 66.04,31.62 ICSP.6 66.04,30.42 67.63,28.83 67.63,17.72 I2C.2
  Bottom 0.813: v18.8,30.48 v24.38,30.48 v31.88,30.48 v32.77,30.48
VIN
  Top 1.27: J8.+ 10.92,2.92 12.45,4.45 12.45,6.22 D1.+
VIN_DC  (via drill 0.3)
  Top 0.61: 22.1,12.19 22.1,12.45 24,14.35 28.45,14.35 29.59,15.49 29.59,16.64 R9.1
  Top 0.813: C11.+ 22.1,12.19
  Top 1.27: U4.3 12.57,13.34 D1.- 14.73,10.67 C10.1 v18.16,10.41 v19.05,10.41 v19.94,10.41 20.7,10.41 C11.+
  Bottom 0.813: v18.16,10.41 v19.05,10.41 v19.94,10.41 21.97,10.41 24.38,8 24.38,2.41 25.84,0.95 44.77,0.95 45.72,1.91 J6.1 J7.1
XB_RST  (via drill 0.3)
  Top 0.305: v15.11,29.15 15.11,34.04 14.35,34.8 v13.08,34.8
  Bottom 0.305: XB_RST.P$1 5.71,51.82 5.71,43.81 6.35,43.18 9.53,43.18 13.08,39.62 v13.08,34.8 | U6.5 15.74,23.38 15.11,24 v15.11,29.15
XB_RX  (via drill 0.3)
  Top 0.305: v63.5,22.23 66.67,22.23 67.5,23.05 67.5,32.19 66.67,33.02 64.77,33.02 63.88,33.91 63.88,37.47 65.02,38.61 v65.66,38.61 | v27.56,28.32 Q1.3 26.8,29.34 26.29,29.84 R17.1
  Bottom 0.305: 60.07,46.74 SERIAL_SELECT.CH1A 58.55,45.21 58.55,40.51 59.05,40.01 61.59,40.01 62.87,41.27 62.87,41.53 SERIAL_SELECT.CH2B 62.99,41.27 v65.66,38.61 | v63.5,22.23 58.55,22.23 50.29,13.97 43.31,13.97 28.96,28.32 v27.56,28.32
XB_RXD  (via drill 0.3)
  Top 0.305: U6.3 11.68,24.38 12.06,24.77 20.32,24.77 v20.95,25.4
  Top 0.406: v27.69,26.16 27.75,26.22 Q1.2 29.02,28.32 R20.2
  Bottom 0.305: v20.95,25.4 26.92,25.4 27.3,25.78
  Bottom 0.406: v27.69,26.16 27.3,25.78
XB_TX  (via drill 0.3)
  Top 0.305: v57.15,24.13 59.69,26.67 60.96,26.67 62.04,27.75 62.04,32.89 63.25,34.1 63.25,38.16 65.15,40.07 65.15,44.07 v64.77,44.45 | v24.26,29.21 24.13,29.08 Q2.3 22.1,29.08 21.72,29.46 21.72,30.1 R18.1
  Bottom 0.305: v57.15,24.13 48.26,15.24 44.7,15.24 30.73,29.21 v24.26,29.21 | SERIAL_SELECT.CH1B 60.2,41.53 61.47,42.8 63.88,42.8 64.64,43.56 64.64,44.32 v64.77,44.45 64.77,44.83 SERIAL_SELECT.CH2A
XB_TXD  (via drill 0.3)
  Top 0.305: U6.2 9.64,25.27 10.16,25.78 17.53,25.78 v18.67,26.92
  Top 0.406: Q2.2 23.68,27.24 v24.51,28.07 | v18.67,26.92 R19.2
  Bottom 0.406: v24.51,28.07 23.37,26.92 v18.67,26.92
XTAL1
  Top 0.305: U2.7 49.63,32.35 50.16,32.89 50.16,34.92 49.91,35.18 C7.2 49.78,36.96 49.78,38.35 50.67,39.24 X1.2
XTAL2
  Top 0.305: U2.8 49.53,33.3 49.53,33.66 47.37,35.81 C8.2 47.12,37.08 47.12,39.12 45.85,40.39 X1.1

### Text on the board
tPlace: PB | PD | 1 | 1 | 1 | 1 | 9 | 8 | 7 | 6 | 5 | 4 | 3 | 2 | 1 | 0 | AREF | GND | 3 | 2 | 1 | 0 | MCU | DIGITAL | PWM | PWM | PWM | USB | VCC | FT_RX | FT_TX | SCL | SDA | 7 | VCC | GND | ADC | ANALOG | 6 | 7 | RST | 3V3 | 5V | GND | VIN | 0 | 1 | 2 | 3 | 4 | 5
bPlace: Crowduino | V1.1 2013/04/11 | www.elecrow.com | PD[0:7] | PB[0:5] | PC[0:5] | PIN | 0 | 1 | 2 | 3 | 4 | 5 | 6 | 7 | 8 | 9 | 10 | 11 | 12 | 13 | 14 | 15 | 16 | 17 | 18 | 19 | FUNCTION | RXD/PCINT16 | TXD/PCINT17 | INT0 | INT1/0C2B | XCK/T0 | 0C0B/T1 | 0C0A/AIN0 | AIN1 | ICP1 | OC1A | SS/0C1B | MOSI/OC2A | MISO | SCK | ADC0 | ADC1 | ADC2 | ADC3 | ADC4/SDA | ADC5/SCL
